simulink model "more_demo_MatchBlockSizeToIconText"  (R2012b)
settings: Solver=ode45  SolverMode=SingleTasking  StartTime=0.0  StopTime=10.0  RelTol=1e-3
model workspace (MAT data in the model file):
  LongConstantName = 0
  ShortConst = 0

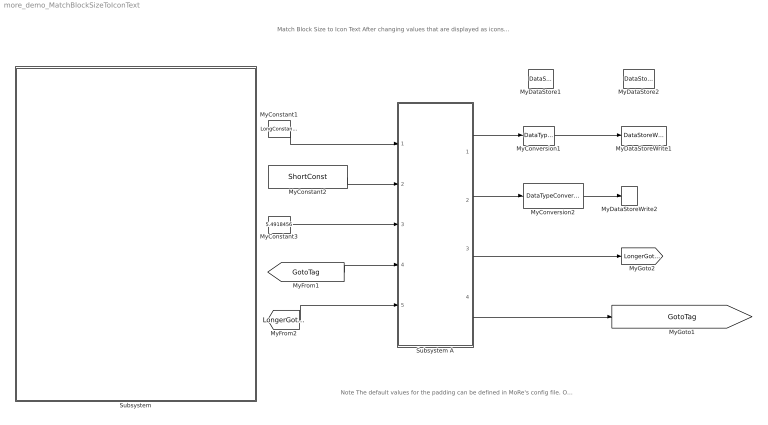
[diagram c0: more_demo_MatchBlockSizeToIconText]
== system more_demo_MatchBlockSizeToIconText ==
  note: Match Block Size to Icon Text After changing values that are displayed as icons on blocks, the blocks might be too big or too small for the icon text. The "Match Blocks to Icon Text" action resizes blocks to match the text displayed on their icon.
  note: Note The default values for the padding can be defined in MoRe's config file. Open the config file via the "Preferences" section of the MoRe menu.
  MyConstant1 : Constant  Value=LongConstantName
  MyConstant2 : Constant  Value=ShortConst
  MyConstant3 : Constant  Value=5.4918456
  MyConversion1 : DataTypeConversion
  MyConversion2 : DataTypeConversion
  MyDataStore1 : DataStoreMemory  DataStoreName=Store  ReadBeforeWriteMsg=warning  WriteAfterWriteMsg=warning  WriteAfterReadMsg=warning
  MyDataStore2 : DataStoreMemory  DataStoreName=LongerStoreName  ReadBeforeWriteMsg=warning  WriteAfterWriteMsg=warning  WriteAfterReadMsg=warning
  MyDataStoreWrite1 : DataStoreWrite  DataStoreName=Store
  MyDataStoreWrite2 : DataStoreWrite  DataStoreName=LongerStoreName
  Subsystem : Subsystem
  Subsystem A : Subsystem
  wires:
  Subsystem A/2(Result2) -> MyConversion2/1
  Subsystem A/1(Result1) -> MyConversion1/1
  MyConversion1/1 -> MyDataStoreWrite1/1
  MyConversion2/1 -> MyDataStoreWrite2/1
  MyConstant1/1 -> Subsystem A/1(MySig1)
  MyConstant2/1 -> Subsystem A/2("MySig2 ")
  MyConstant3/1 -> Subsystem A/3(MySig3)
  [GotoTag] -> Subsystem A/4(MySi4)
  [LongerGotoTag] -> Subsystem A/5(MySig5)
  Subsystem A/3(Result3) -> [LongerGotoTag]
  Subsystem A/4(Result4) -> [GotoTag]

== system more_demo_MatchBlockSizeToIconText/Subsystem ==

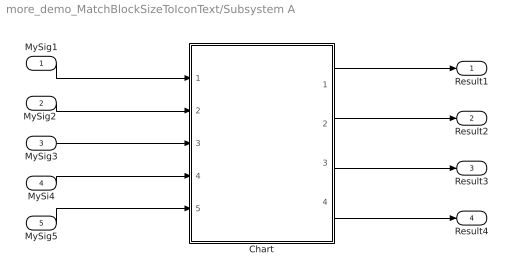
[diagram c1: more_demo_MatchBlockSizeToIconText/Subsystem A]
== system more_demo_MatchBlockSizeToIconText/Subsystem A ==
  MySig1 : Inport
  "MySig2 " : Inport  Port=2
  MySig3 : Inport  Port=3
  MySi4 : Inport  Port=4
  MySig5 : Inport  Port=5
  Chart : Stateflow chart  TreatAsAtomicUnit=on
  Result1 : Outport
  Result2 : Outport  Port=2
  Result3 : Outport  Port=3
  Result4 : Outport  Port=4
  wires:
  MySig1/1 -> Chart/1(MySig1)
  "MySig2 "/1 -> Chart/2(MySig2)
  Chart/4(Result4) -> Result4/1
  Chart/3(Result3) -> Result3/1
  Chart/2(Result2) -> Result2/1
  Chart/1(Result1) -> Result1/1
  MySig3/1 -> Chart/3(MySig3)
  MySi4/1 -> Chart/4(MySig4)
  MySig5/1 -> Chart/5(MySig5)
